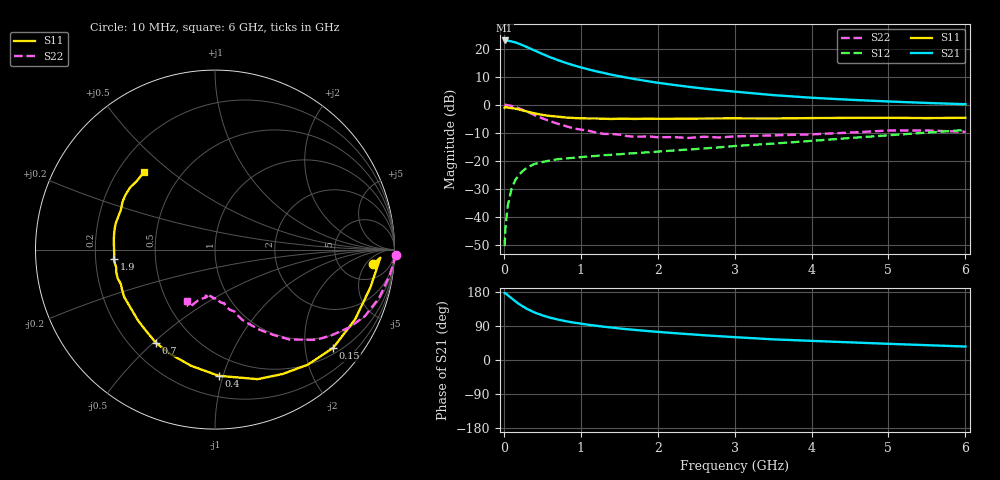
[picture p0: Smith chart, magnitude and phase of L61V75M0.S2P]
!  INFINEON TECHNOLOGIES Small Signal Semiconductors
! BFR380L3 , Si-NPN RF-Transistor in TSLP-3-1
!  Vce=1.75 V,  Ic=5 mA
! Common Emitter S-Parameters:  07. March 2005
#  GHz  S  MA  R  50
! f  S11  S21  S12  S22
! GHz  Mag  Ang  Mag  Ang  Mag  Ang  Mag  Ang
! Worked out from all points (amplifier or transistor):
!   36 points, 10 MHz to 6 GHz, reference 50 ohm
!   highest |S21| = 23.0 dB at 10 MHz (marker M1)
!   |S21| within 3 dB of that: start of sweep to 351.4 MHz
!   unconditionally stable (mu >= 1): 2.368 GHz to 4.777 GHz
!   at 250 MHz: K = 0.17, MSG = 22.4 dB, |S12| = -23.5 dB
!   at 1.4 GHz: K = 0.76, MSG = 14.3 dB, |S12| = -17.9 dB
!   at 6 GHz: K = 0.95, MSG = 4.6 dB, |S12| = -9.0 dB
!   S11 on the Smith chart (normalised r, x): 10 MHz: 11, -8; 150 MHz: 0.64, -2.63; 400 MHz: 0.35, -0.97; 700 MHz: 0.31, -0.51; 1.9 GHz: 0.28, -0.04; 6 GHz: 0.31, +0.40
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0.01  0.8847 -5.1  14.07 176.6  0.003 87.2  1.011 -1.7
0.02  0.9224 -2.8  14.07 176.8  0.0061 89.8  1 -3.6
0.05  0.8911 -13.7  13.93 171.2  0.0155 82.3  0.9838 -8.3
0.1  0.872 -26.5  13.51 162.9  0.0319 77.0  0.9532 -16.4
0.15  0.8563 -39.7  13 154.8  0.0458 69.6  0.9136 -24.0
0.2  0.8238 -51.1  12.25 147.3  0.0568 64.3  0.8635 -30.2
0.25  0.7891 -61.4  11.5 141.1  0.0666 59.6  0.8053 -36.4
0.3  0.7599 -71.8  10.71 135.0  0.0756 56.0  0.7563 -41.6
0.4  0.7034 -88.3  9.31 125.3  0.0882 49.7  0.6529 -50.2
0.5  0.661 -101.6  8.096 117.9  0.0951 45.6  0.5739 -55.8
0.6  0.6325 -113.3  7.081 111.6  0.1016 42.9  0.5112 -60.9
0.7  0.6155 -122.1  6.292 106.9  0.1069 41.2  0.4598 -65.0
0.9  0.5828 -137.6  5.098 99.0  0.1131 39.7  0.3812 -71.5
1.1  0.5703 -147.7  4.287 92.9  0.12 40.0  0.3441 -76.4
1.4  0.5584 -159.8  3.443 85.7  0.1279 41.1  0.3014 -81.7
1.9  0.5653 -174.7  2.597 75.9  0.1426 44.7  0.2723 -91.8
2.2  0.5629 178.8  2.275 71.1  0.1527 47.1  0.2658 -93.5
2.8  0.5714 167.6  1.826 62.8  0.1741 51.6  0.2612 -101.4
3.5  0.5691 157.3  1.49 54.5  0.2031 54.5  0.2849 -105.9
4.5  0.5843 148.8  1.23 46.6  0.2553 58.5  0.3193 -110.9
5.5  0.5795 138.8  1.079 39.1  0.3191 58.7  0.3482 -115.7
6  0.5863 132.6  1.025 35.5  0.3551 57.8  0.3296 -118.7
